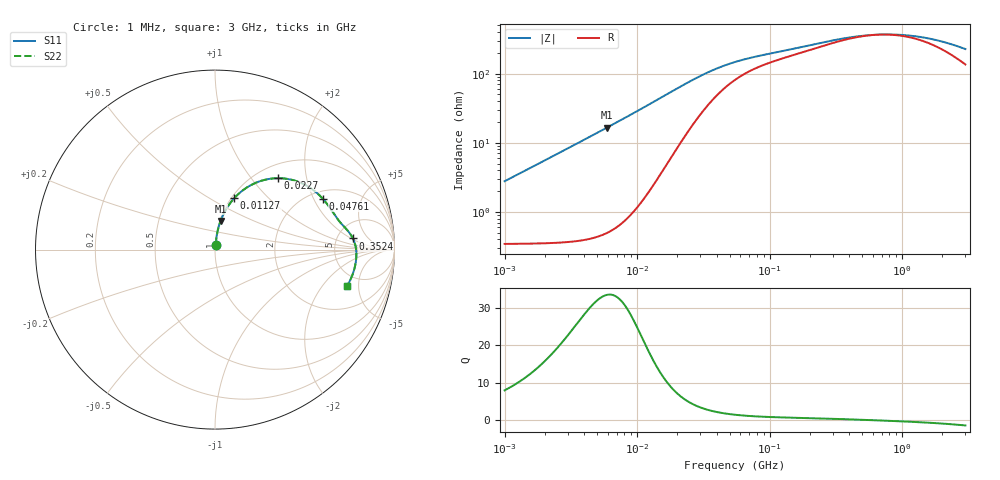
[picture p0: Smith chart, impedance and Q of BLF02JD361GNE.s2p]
! BLF02JD361GNE
# Hz S RI R 50
!Freq.(Hz) S11(Real) S11(Imag) S21(Real) S21(Imag) S12(Real) S12(Imag) S22(Real) S22(Imag)
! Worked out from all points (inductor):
!   401 points, 1 MHz to 3 GHz, reference 50 ohm
!   read as one part in series: L = 439 nH near 1.041 MHz
!   highest Q = 33.5 at 5.938 MHz (marker M1), where L = 446 nH
!   self-resonance near 670.9 MHz
!   S11 on the Smith chart (normalised r, x): 1 MHz: 1.01, +0.06; 11.27 MHz: 1.03, +0.65; 22.7 MHz: 1.24, +1.38; 47.61 MHz: 2.32, +2.36; 352.4 MHz: 7.06, +2.15; 3 GHz: 3.72, -3.65
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1000000  0.00417 0.0273  0.9958 -0.0273  0.9958 -0.0273  0.00417 0.0273
2097170  0.00681 0.0573  0.9932 -0.0573  0.9932 -0.0573  0.00681 0.0573
3823119  0.0148 0.1041  0.9852 -0.1041  0.9852 -0.1041  0.0148 0.1041
5938264  0.0314 0.1602  0.9686 -0.1602  0.9686 -0.1602  0.0314 0.1602
8513927  0.0621 0.2251  0.9379 -0.2251  0.9379 -0.2251  0.0621 0.2251
1.126754e7  0.1073 0.2866  0.8927 -0.2866  0.8927 -0.2866  0.1073 0.2866
1.461624e7  0.1757 0.3449  0.8243 -0.3449  0.8243 -0.3449  0.1757 0.3449
1.858443e7  0.2649 0.3855  0.7351 -0.3855  0.7351 -0.3855  0.2649 0.3855
2.270269e7  0.3524 0.3978  0.6476 -0.3978  0.6476 -0.3978  0.3524 0.3978
2.718395e7  0.431 0.3881  0.569 -0.3881  0.569 -0.3881  0.431 0.3881
3.320783e7  0.5071 0.3581  0.4929 -0.3581  0.4929 -0.3581  0.5071 0.3581
4.761141e7  0.6 0.284  0.4 -0.284  0.4 -0.284  0.6 0.284
5.477226e7  0.6229 0.2564  0.3771 -0.2564  0.3771 -0.2564  0.6229 0.2564
9.216659e7  0.6762 0.1795  0.3238 -0.1795  0.3238 -0.1795  0.6762 0.1795
2.094008e8  0.7374 0.1078  0.2626 -0.1078  0.2626 -0.1078  0.7374 0.1078
3.523638e8  0.7684 0.0619  0.2316 -0.0619  0.2316 -0.0619  0.7684 0.0619
5.364635e8  0.7825 0.022  0.2175 -0.022  0.2175 -0.022  0.7825 0.022
8.005644e8  0.7876 -0.0179  0.2124 0.0179  0.2124 0.0179  0.7876 -0.0179
1.10276e9  0.7865 -0.0528  0.2135 0.0528  0.2135 0.0528  0.7865 -0.0528
1.519029e9  0.7801 -0.0928  0.2199 0.0928  0.2199 0.0928  0.7801 -0.0928
2.050964e9  0.7671 -0.1372  0.2329 0.1372  0.2329 0.1372  0.7671 -0.1372
3e9  0.7347 -0.2048  0.2653 0.2048  0.2653 0.2048  0.7347 -0.2048
